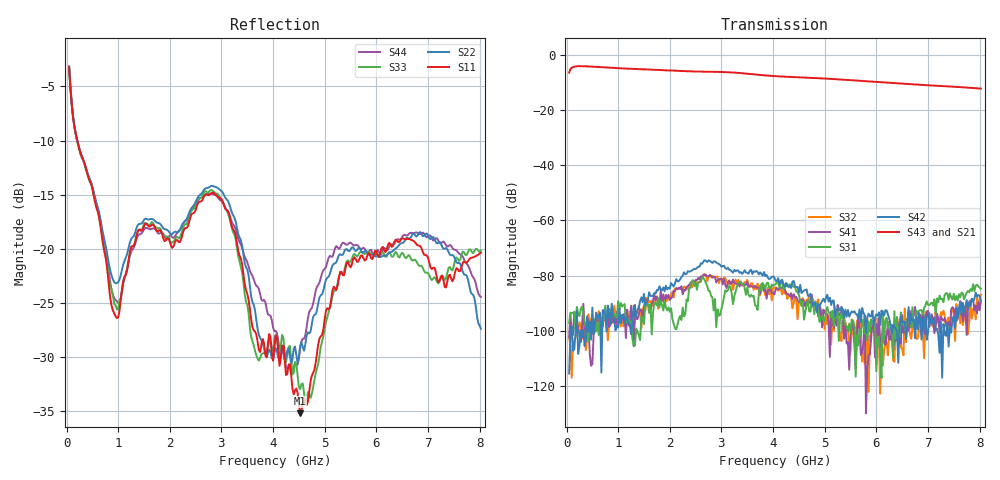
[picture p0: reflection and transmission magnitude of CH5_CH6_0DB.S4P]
!Agilent Technologies,E5071C,MY46316741,A.11.02
!Date: Mon Jun 01 10:38:48 2026
!Data & Calibration Information:
!1:CH5 INPUT 2:CH5 OUTPUT 3:CH6 INPUT 4:CH6 OUTPUT
!Freq	S11:SOLT4(ON)	S12:SOLT4(ON)	S13:SOLT4(ON)	S14:SOLT4(ON)
!	S21:SOLT4(ON)	S22:SOLT4(ON)	S23:SOLT4(ON)	S24:SOLT4(ON)
!	S31:SOLT4(ON)	S32:SOLT4(ON)	S33:SOLT4(ON)	S34:SOLT4(ON)
!	S41:SOLT4(ON)	S42:SOLT4(ON)	S43:SOLT4(ON)	S44:SOLT4(ON)
!PortZ  Port1:50+j0  Port2:50+j0  Port3:50+j0  Port4:50+j0
!Above PortZ is port z conversion or system Z0 setting when saving the data.
!When reading, reference impedance value at option line is always used.
# Hz S dB R 50
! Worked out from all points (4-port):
!   320 points, 50 MHz to 8.025 GHz, reference 50 ohm
!   strongest paths, dB at 50 MHz, 2.05 GHz, 4.05 GHz, 6.05 GHz, 8.025 GHz:
!     S43: -6.5, -5.7, -7.8, -9.9, -12.2
!     S21: -6.5, -5.9, -8.0, -10.1, -12.6
!     S42: -115.5, -83.3, -81.9, -93.3, -89.1
!     S31: -97.2, -95.7, -83.2, -102.1, -84.8
!     S41: -102.5, -87.6, -85.0, -95.3, -89.4
!     S32: -102.1, -85.9, -84.2, -100.7, -86.9
!   lowest |S11| = -35.2 dB at 4.525 GHz (marker M1), VSWR 1.04, Z = 49.9 - j1.74 ohm
!   |S11| at or under -10 dB: 209.1 MHz to end of sweep
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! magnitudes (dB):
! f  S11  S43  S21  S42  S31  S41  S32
! 50 MHz  -3.2  -6.5  -6.5  -115.5  -97.2  -102.5  -102.1
! 950 MHz  -26.2  -4.8  -5.0  -99.9  -94.5  -98.9  -94.7
! 2.85 GHz  -14.8  -6.2  -6.4  -74.9  -92.6  -80.5  -80.4
! 3.875 GHz  -30.0  -7.5  -7.7  -79.7  -82.8  -88.4  -86.5
! 4.525 GHz  -35.2  -8.2  -8.4  -83.4  -89.3  -89.1  -89.5
! 5.45 GHz  -21.2  -9.1  -9.3  -92.5  -100.1  -104.2  -98.7
! 8.025 GHz  -20.3  -12.2  -12.6  -89.1  -84.8  -89.4  -86.9
